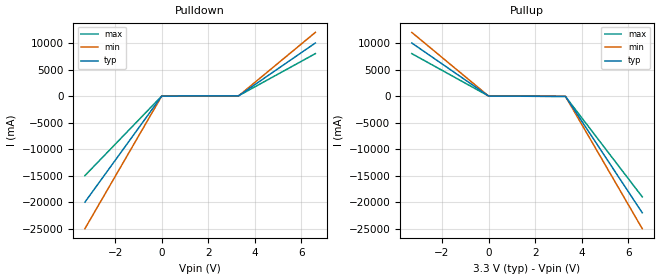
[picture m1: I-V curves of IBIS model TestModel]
[IBIS Ver]   3.2
[File Name]   bug42.ibs
[File Rev]   0.0
[Date]   09-May-2000
[Source]   File created from specification
[Disclaimer]
   (C) Copyright 2000 Intel Corp.
   All rights reserved
   This model is for demonstration purposes only,
   to show Vinh and Vinl
[Component]   GENERIC_IBIS
[Manufacturer]   Intel Corp.
[Package]
|   typ   min   max
R_pkg   6.0mO   5.0mO   7.0mO
L_pkg   5.0nH   2.0nH   8.0nH
C_pkg   1.0pF   0.5pF   1.5pF
[Pin]   signal_name   model_name   R_pin   L_pin   C_pin
   1   TestSignal   TestModel
| Models and submodels in the file (1): TestModel (Output)
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[Model]   TestModel
Model_type   Output
Polarity   Non-Inverting
Vinh = 1
Vinl = .2
Cref = 10.0pF
C_comp   5.00pF   4.00pF   6.00pF
[Temperature Range]   27.00   100.00   0.00
[Voltage Range]   3.30V   3.00V   3.60V
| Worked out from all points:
|   slope of the pulldown table from 0 to 0.495 V, typ, clamps not added: 82.5 ohm
|   slope of the pullup table from 0 to 0.495 V, typ, clamps not added: 50.8 ohm
[Pulldown]
| voltage   I(typ)   I(min)   I(max)
-3.3V     -20A       -25A       -15A
0V        0A         -5nA       5nA
3.3V      40mA       32mA       48mA
6.6V      10A        12A        8A
[Pullup]
| voltage   I(typ)   I(min)   I(max)
-3.3V     10A        12A        8A
0V        0A         -300nA     300nA
3.3V      -65mA      -40mA      -80mA
6.6V      -22A       -25A       -19A
[Ramp]
| variable   typ   min   max
dV/dt_r   0.35/1.6n   0.25/1.8n   0.45/1.5n
dV/dt_f   0.35/1.6n   0.25/1.8n   0.45/1.5n
R_load = 50.000
